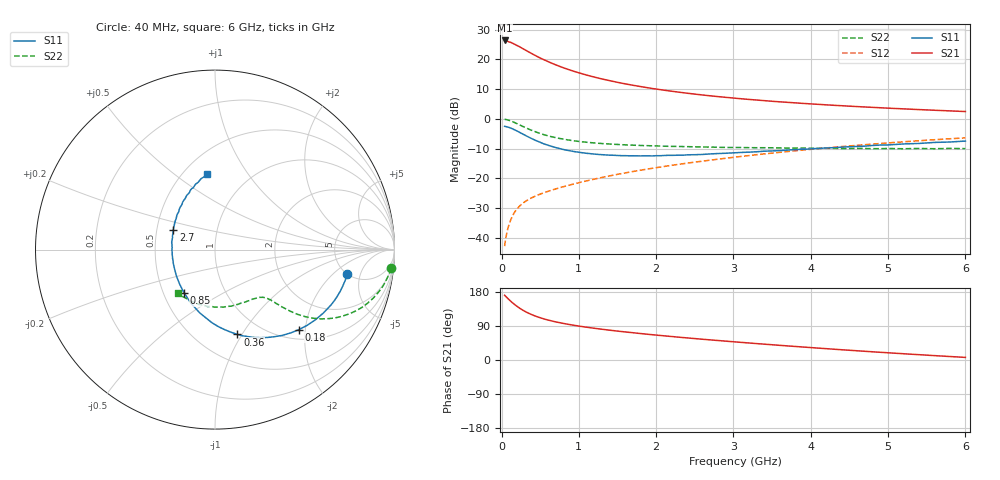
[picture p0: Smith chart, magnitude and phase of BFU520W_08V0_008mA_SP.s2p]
! Filename:  P:\Prog\Test\Noise\ATS_data\Testdata_Net\Run2\BFU520W_APM2013_06_A05_08p0V_008mA_SP_CM01_D.s2p
! Date/Time: Tue 26/Mar/2013 18:01:42
! BFU520W_APM2013_06_A05_08p0V_1to20mA_SP_CM01_Bias5_R.s2p
! MDIF S-parameter v. bias file
! BFU520W_APM2013_06_A05_08p0V_1to20mA_SP_CM01
! Date/time Thu Mar 21 15:28:29 2013
! VAR V_out= 8.0000
! VAR I_out= 7.9950
! VAR V_in= 0.8259
! VAR I_in= 0.0873
! Device data file deembeded for feedlines and parallel
! Original file: \Run2\BFU520W_APM2013_06_A05_08p0V_008mA_SP_CM01_R.s2p
! Feed-files: PR019V01_070313_Feed1.s2p, PR019V01_070313_Feed2.s2p
! Parallel-file: PR019V01_070313_Par.s2p
# MHz S MA R 50
!  Freq-MHz  S11-mag  S11-arg  S21-mag  S21-arg  S12-mag  S12-arg  S22-mag  S22-arg
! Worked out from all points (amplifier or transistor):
!   98 points, 40 MHz to 6 GHz, reference 50 ohm
!   highest |S21| = 26.3 dB at 40 MHz (marker M1)
!   |S21| within 3 dB of that: start of sweep to 293 MHz
!   unconditionally stable (mu >= 1): 1.59 GHz to 2.796 GHz
!   at 300 MHz: K = 0.44, MSG = 25.6 dB, |S12| = -27.9 dB
!   at 1.6 GHz: K = 1.00, MAG = 14.8 dB, |S12| = -18.1 dB
!   at 6 GHz: K = 0.87, MSG = 4.4 dB, |S12| = -6.4 dB
!   S11 on the Smith chart (normalised r, x): 40 MHz: 5.00, -3.11; 180 MHz: 1.21, -1.85; 360 MHz: 0.77, -0.95; 850 MHz: 0.64, -0.34; 2.7 GHz: 0.61, +0.15; 6 GHz: 0.65, +0.67
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40  0.7496 -10.4  20.77 170.8  0.007286 84.6  0.9848 -6.0
50  0.7461 -12.9  20.76 168.7  0.008997 83.3  0.9813 -7.5
80  0.7299 -20.7  20.09 162.6  0.01405 79.8  0.96 -11.8
120  0.6993 -30.4  19.27 154.9  0.02029 75.5  0.9227 -17.0
140  0.6826 -35.0  18.75 151.3  0.02313 73.6  0.9008 -19.4
180  0.646 -43.6  17.64 144.8  0.02838 70.2  0.855 -23.6
220  0.6077 -51.9  16.63 138.7  0.03288 67.7  0.8087 -27.0
260  0.5706 -59.1  15.55 133.4  0.03688 65.6  0.7642 -29.9
320  0.5184 -69.3  14.07 126.5  0.04207 63.4  0.7032 -33.3
360  0.4887 -75.2  13.15 122.5  0.04514 62.4  0.6674 -34.9
440  0.4361 -86.0  11.57 115.8  0.05071 61.3  0.6068 -37.3
550  0.3798 -98.6  9.841 108.3  0.05751 60.9  0.5423 -39.3
700  0.3304 -112.9  8.103 100.7  0.06661 61.4  0.4844 -40.7
850  0.297 -125.2  6.86 94.6  0.07564 62.2  0.4455 -41.5
1050  0.2696 -138.9  5.689 88.0  0.08792 63.4  0.4118 -42.5
1500  0.2429 -163.7  4.115 76.3  0.1171 64.7  0.3722 -45.6
2050  0.2409 174.0  3.101 64.8  0.155 64.5  0.3503 -51.4
2700  0.2581 154.3  2.442 53.1  0.2028 62.6  0.3361 -60.9
3100  0.2732 144.0  2.179 46.5  0.2343 60.8  0.3308 -67.2
4100  0.3203 124.2  1.756 31.3  0.317 54.6  0.3199 -86.5
5200  0.3797 106.8  1.474 16.5  0.4125 45.5  0.3153 -110.9
6000  0.4243 95.8  1.329 6.9  0.4804 38.0  0.3169 -131.0
